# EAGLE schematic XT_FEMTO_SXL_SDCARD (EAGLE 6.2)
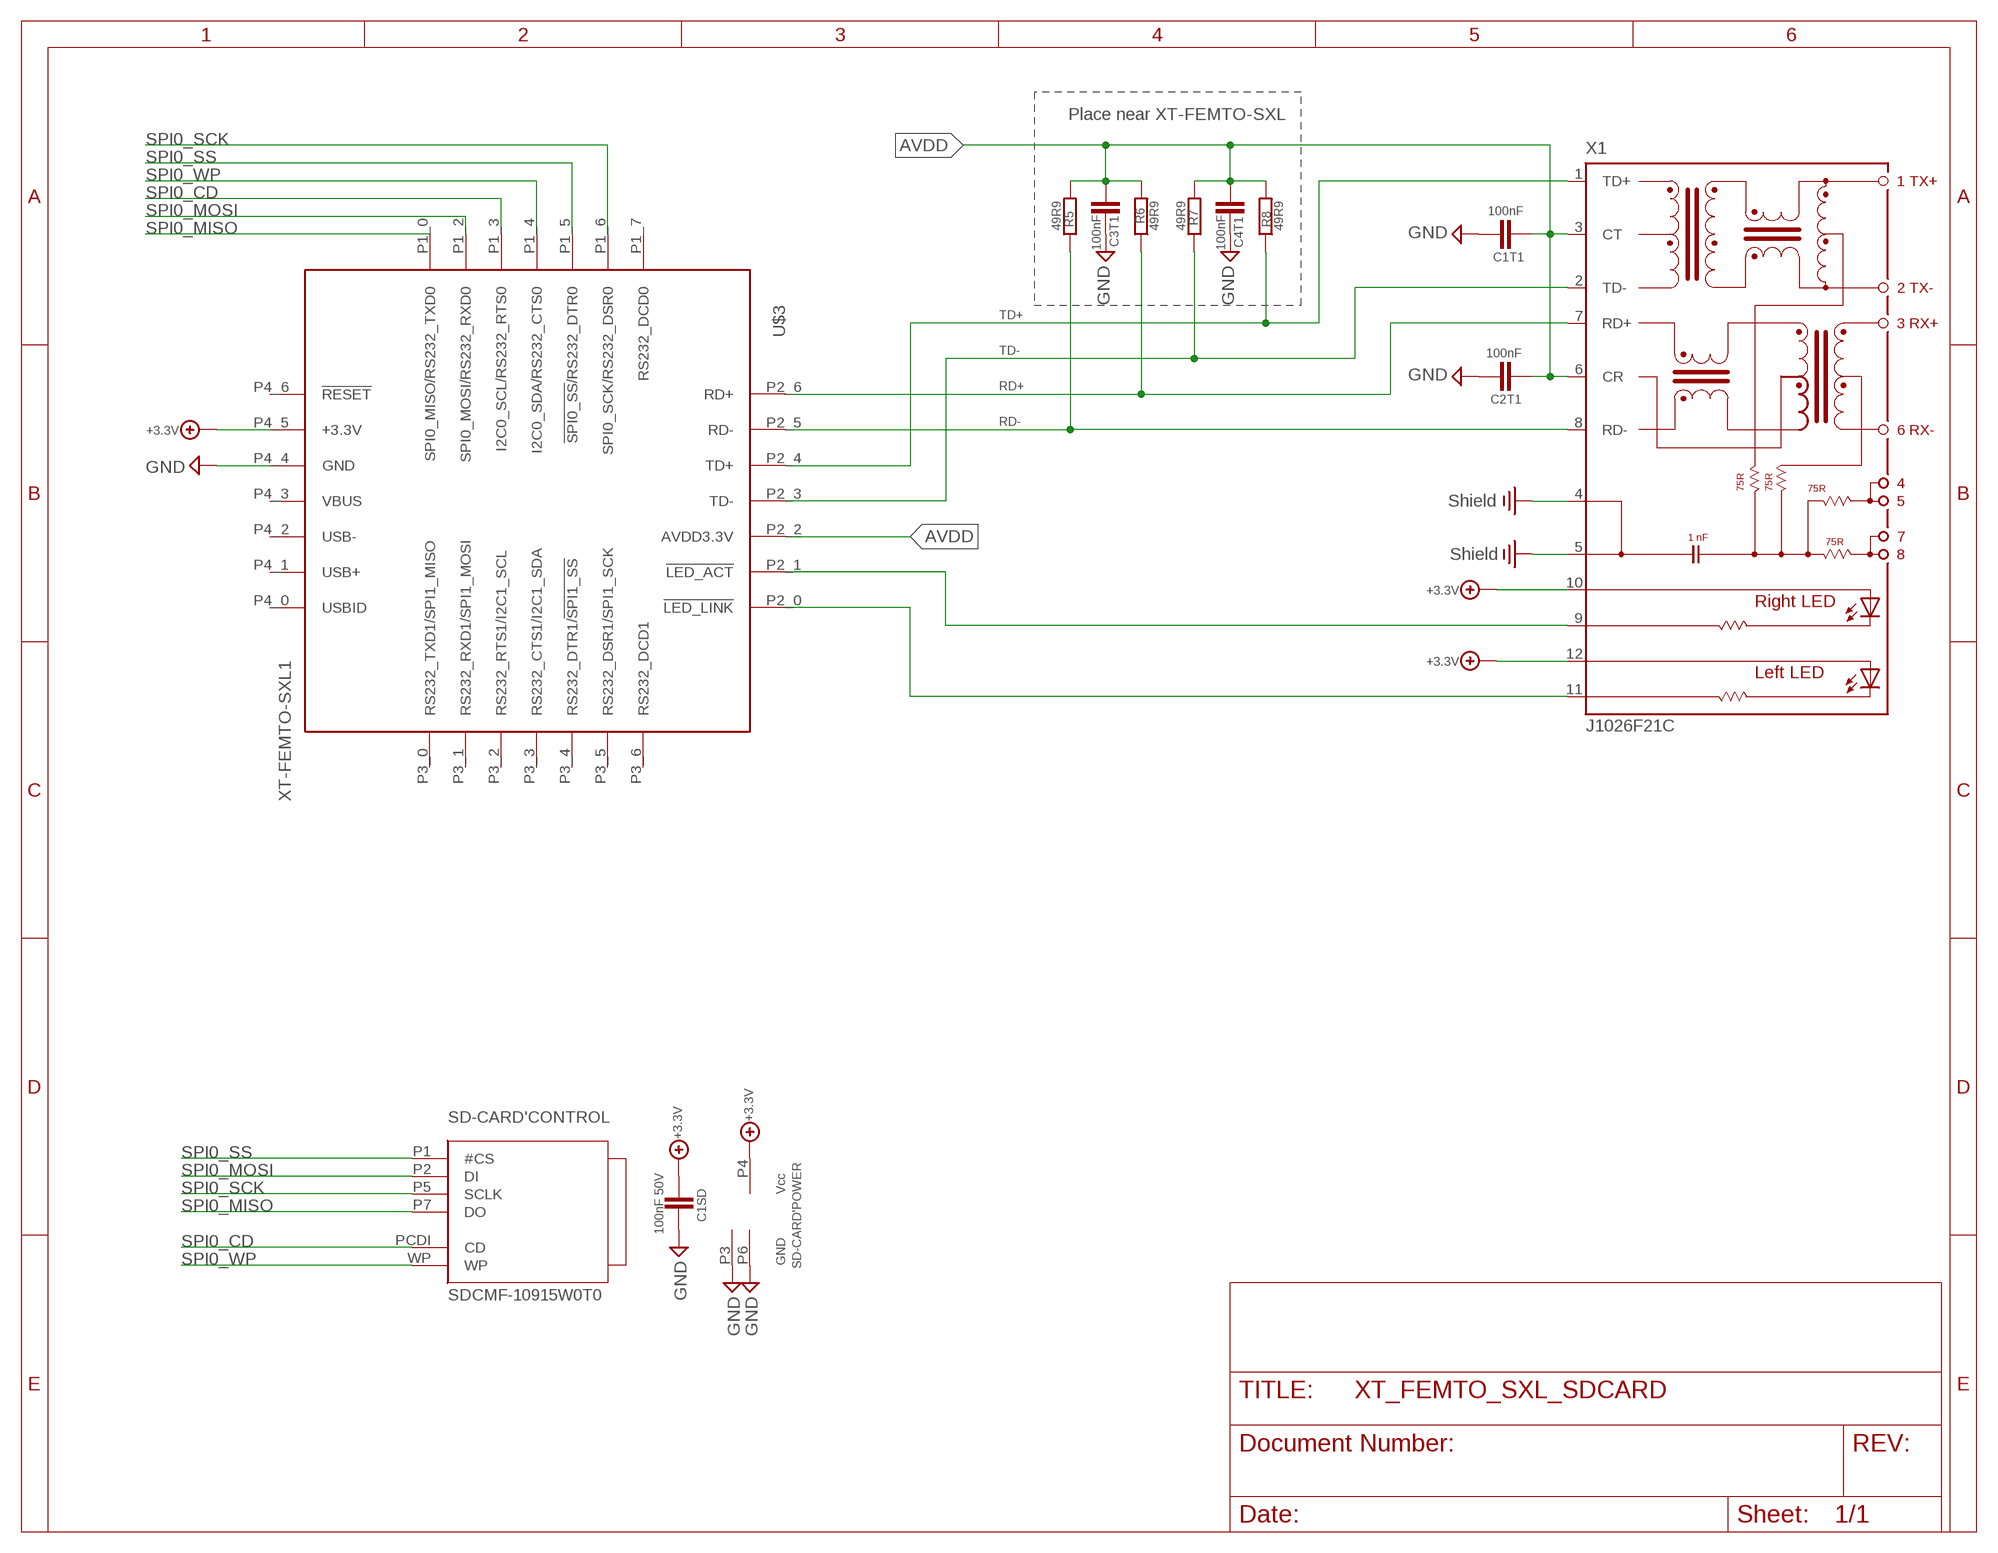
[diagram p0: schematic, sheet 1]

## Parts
C1SD  100nF 50V  CHIP-C-0603  [SMD-0603]
C1T1  100nF  CHIP-C-VTS0402  [R0402_VTS]
C2T1  100nF  CHIP-C-VTS0402  [R0402_VTS]
C3T1  100nF  CHIP-C-VTS0402  [R0402_VTS]
C4T1  100nF  CHIP-C-VTS0402  [R0402_VTS]
R5  49R9  R-EU_R0603  [R0603]
R6  49R9  R-EU_R0603  [R0603]
R7  49R9  R-EU_R0603  [R0603]
R8  49R9  R-EU_R0603  [R0603]
SD-CARD  SDCMF-10915W0T0  SDCMF-109XXW010SDCMF-10915W0T1_SO  [SDCMF-10915W0T1]
U$3  XT-FEMTO-SXL1  [XT-FEMTO-SXL-PIN]
X1  J1026F21C  [J1]

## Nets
+3.3V: C1SD.2 SD-CARD.P4('POWER:VCC) U$3.P4_5(+3.3V) X1.10(A-R) X1.12(A-L)
AVDD: C1T1.1 C2T1.2 C3T1.1 C4T1.2 R5.2 R6.2 R7.2 R8.2 U$3.P2_2(AVDD3.3V) X1.3(CT) X1.6(CR)
GND: C1SD.1 C1T1.2 C2T1.1 C3T1.2 C4T1.1 SD-CARD.P3('POWER:GND) SD-CARD.P6('POWER:GND) U$3.P4_4(GND)
N$3: U$3.P2_1(!LED_ACT) X1.9(C-R)
N$5: U$3.P2_0(!LED_LINK) X1.11(C-L)
PE: X1.4 X1.5 ; supply symbol labelled Shield
RD+: R6.1 U$3.P2_6(RD+) X1.7(RD+)
RD-: R5.1 U$3.P2_5(RD-) X1.8(RD-)
SPI0_CD: SD-CARD.PCDI('CONTROL:CD) U$3.P1_3(I2C0_SCL/RS232_RTS0)
SPI0_MISO: SD-CARD.P7('CONTROL:DO) U$3.P1_0(SPI0_MISO/RS232_TXD0)
SPI0_MOSI: SD-CARD.P2('CONTROL:DI) U$3.P1_2(SPI0_MOSI/RS232_RXD0)
SPI0_SCK: SD-CARD.P5('CONTROL:SCLK) U$3.P1_6(SPI0_SCK/RS232_DSR0)
SPI0_SS: SD-CARD.P1('CONTROL:#CS) U$3.P1_5(!SPI0_SS!/RS232_DTR0)
SPI0_WP: SD-CARD.WP('CONTROL:WP) U$3.P1_4(I2C0_SDA/RS232_CTS0)
TD+: R8.1 U$3.P2_4(TD+) X1.1(TD+)
TD-: R7.1 U$3.P2_3(TD-) X1.2(TD-)
Unconnected: U$3.P1_7(RS232_DCD0) U$3.P3_0(RS232_TXD1/SPI1_MISO) U$3.P3_1(RS232_RXD1/SPI1_MOSI) U$3.P3_2(RS232_RTS1/I2C1_SCL) U$3.P3_3(RS232_CTS1/I2C1_SDA) U$3.P3_4(RS232_DTR1/!SPI1_SS!) U$3.P3_5(RS232_DSR1/SPI1_SCK) U$3.P3_6(RS232_DCD1) U$3.P4_0(USBID) U$3.P4_1(USB+) U$3.P4_2(USB-) U$3.P4_3(VBUS) U$3.P4_6(!RESET)

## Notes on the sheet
- Place near XT-FEMTO-SXL

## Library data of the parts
C1SD C1T1 C2T1 C3T1 C4T1 = mea-lib:CHIP-C-?: Chip capacitance
R5-R8 = rcl:R-EU_: RESISTOR, European symbol
SD-CARD = sdcards:SDCMF-109XXW010: KingFont SD-CARD SDCMF-109XXW010 SPI -MODE
U$3 = ak-devices:XT-FEMTO-SXL: AK-NORD XT-FEMTO-SXL
X1 = con-pulse:J1026F: PULSEJACK (TM) 1x1 Tab-UP RJ45 10/100 Base-TX RJ45 1x1 Tab-UP with LEDs 8-pin (J1 series) and 6-pin (JP series) integrated magnetics connector, designed to support applications, such as ADSL modems, LAN-on-Motherboard, and Hub and Switches. Source: www.pulseeng.com .. PulseJack-J402.pdf; OC_FARNELL: unknown; OC_NEWARK: unknown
